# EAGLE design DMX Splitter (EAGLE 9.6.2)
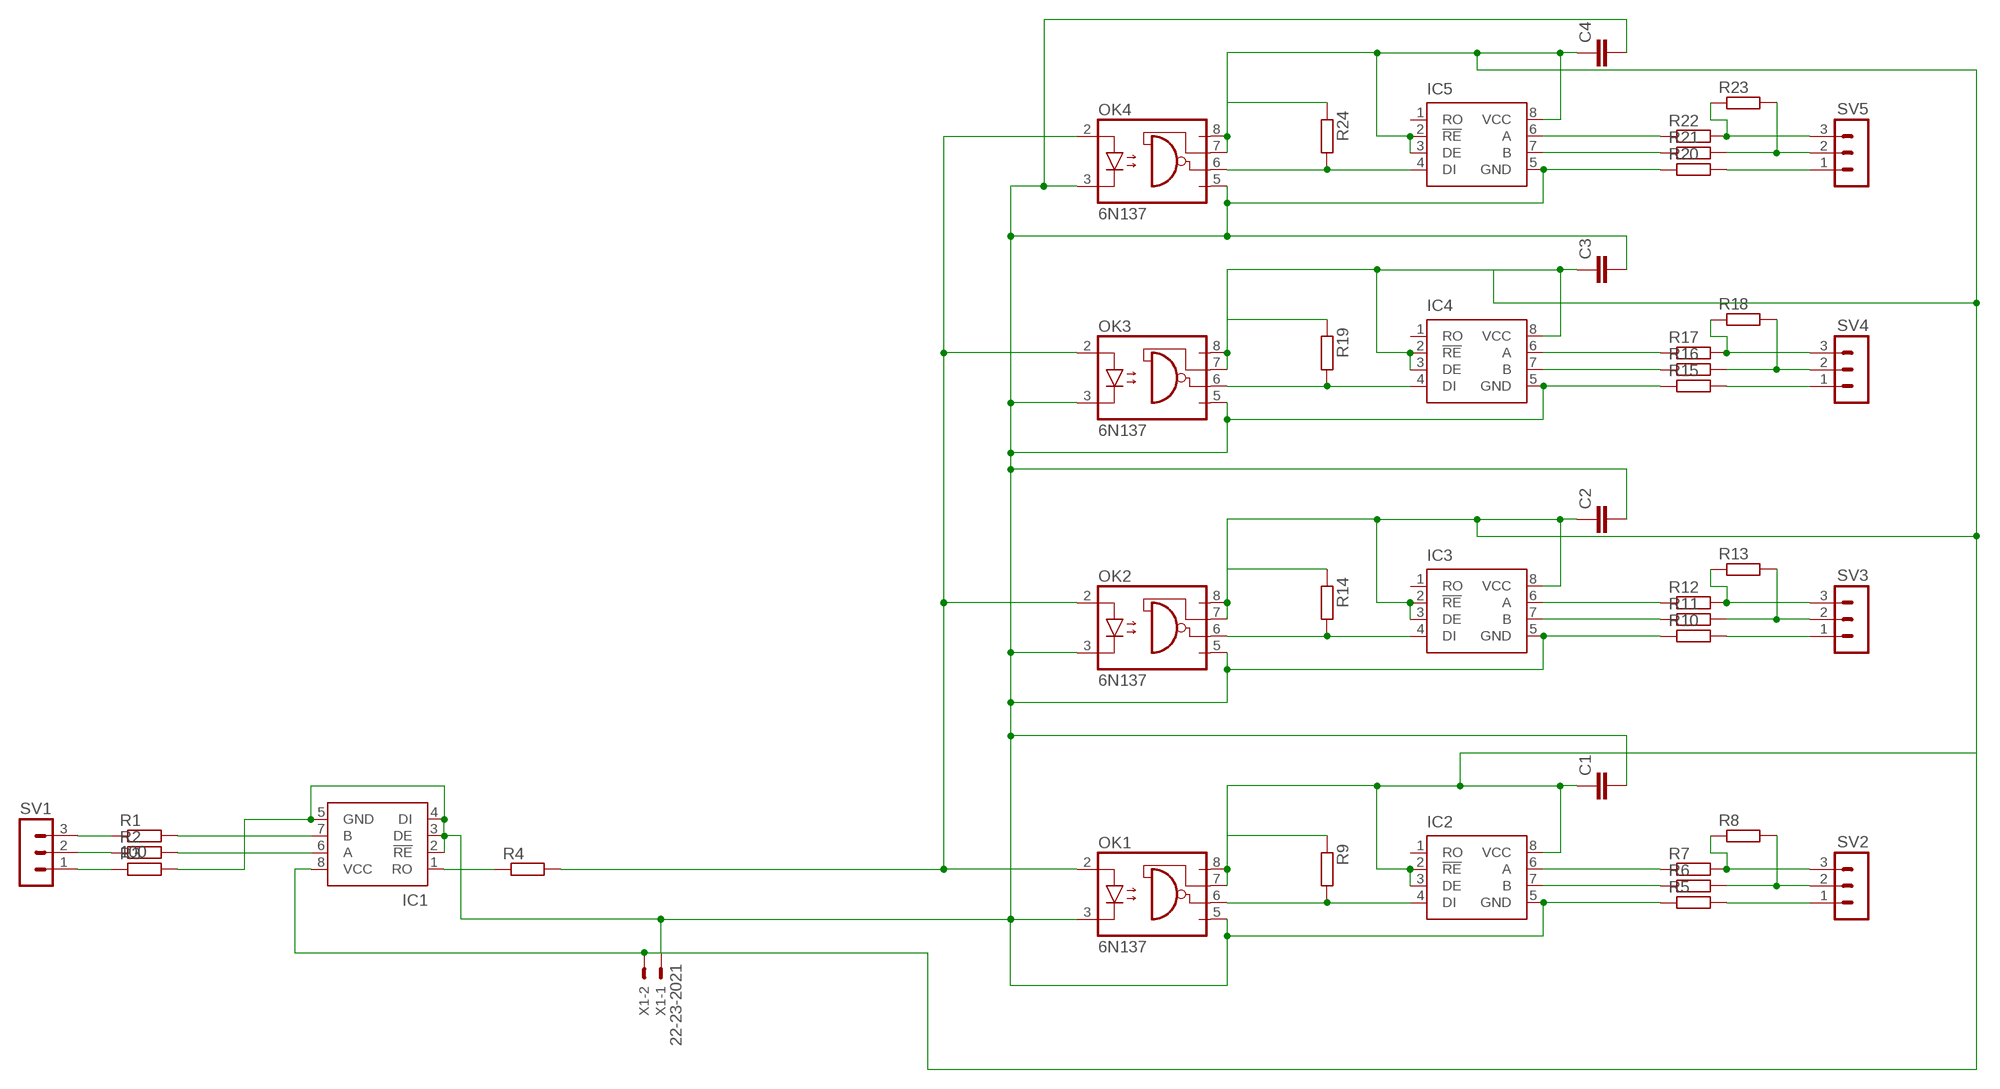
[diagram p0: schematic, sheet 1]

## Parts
C1  C-EUC025_050-024X070  [C025_050-024X070]
C2  C-EUC025_050-024X070  [C025_050-024X070]
C3  C-EUC025_050-024X070  [C025_050-024X070]
C4  C-EUC025_050-024X070  [C025_050-024X070]
IC1  LTC485N  [DIL08]
IC2  LTC485N  [DIL08]
IC3  LTC485N  [DIL08]
IC4  LTC485N  [DIL08]
IC5  LTC485N  [DIL08]
OK1  6N137  [DIL08]
OK2  6N137  [DIL08]
OK3  6N137  [DIL08]
OK4  6N137  [DIL08]
R1  100  R-EU_0207/2V  [0207/2V]
R2  R-EU_0207/2V  [0207/2V]
R3  R-EU_0207/2V  [0207/2V]
R4  R-EU_0207/2V  [0207/2V]
R5  R-EU_0207/2V  [0207/2V]
R6  R-EU_0207/2V  [0207/2V]
R7  R-EU_0207/2V  [0207/2V]
R8  R-EU_0207/2V  [0207/2V]
R9  R-EU_0207/2V  [0207/2V]
R10  R-EU_0207/2V  [0207/2V]
R11  R-EU_0207/2V  [0207/2V]
R12  R-EU_0207/2V  [0207/2V]
R13  R-EU_0207/2V  [0207/2V]
R14  R-EU_0207/2V  [0207/2V]
R15  R-EU_0207/2V  [0207/2V]
R16  R-EU_0207/2V  [0207/2V]
R17  R-EU_0207/2V  [0207/2V]
R18  R-EU_0207/2V  [0207/2V]
R19  R-EU_0207/2V  [0207/2V]
R20  R-EU_0207/2V  [0207/2V]
R21  R-EU_0207/2V  [0207/2V]
R22  R-EU_0207/2V  [0207/2V]
R23  R-EU_0207/2V  [0207/2V]
R24  R-EU_0207/2V  [0207/2V]
SV1  MA03-1  [MA03-1]
SV2  MA03-1  [MA03-1]
SV3  MA03-1  [MA03-1]
SV4  MA03-1  [MA03-1]
SV5  MA03-1  [MA03-1]
X1  22-23-2021  [22-23-2021]

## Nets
N$1: R1.1 SV1.3
N$2: R2.1 SV1.2
N$3: R3.1 SV1.1
N$4: IC1.7(B) R1.2
N$5: IC1.6(A) R2.2
N$7: IC1.1(RO) R4.1
N$9: IC2.4(DI) OK1.6(VO) R9.2
N$11: C1.1 IC2.2(!RE) IC2.3(DE) IC2.8(VCC) OK1.7(VE) OK1.8(VCC) R9.1
N$12: R7.2 R8.1 SV2.3
N$13: IC2.6(A) R7.1
N$14: R6.2 R8.2 SV2.2
N$15: R5.2 SV2.1
N$16: IC2.7(B) R6.1
N$18: IC3.4(DI) OK2.6(VO) R14.2
N$19: C2.1 C3.1 C4.1 IC1.8(VCC) IC3.2(!RE) IC3.3(DE) IC3.8(VCC) IC4.2(!RE) IC4.3(DE) IC4.8(VCC) IC5.2(!RE) IC5.3(DE) IC5.8(VCC) OK2.7(VE) OK2.8(VCC) OK3.7(VE) OK3.8(VCC) OK4.7(VE) OK4.8(VCC) R14.1 R19.1 R24.1 X1.2
N$21: R12.2 R13.1 SV3.3
N$22: IC3.6(A) R12.1
N$23: R11.2 R13.2 SV3.2
N$24: R10.2 SV3.1
N$25: IC3.7(B) R11.1
N$26: IC4.4(DI) OK3.6(VO) R19.2
N$29: R17.2 R18.1 SV4.3
N$30: IC4.6(A) R17.1
N$31: R16.2 R18.2 SV4.2
N$32: R15.2 SV4.1
N$33: IC4.7(B) R16.1
N$34: IC5.4(DI) OK4.6(VO) R24.2
N$37: R22.2 R23.1 SV5.3
N$38: IC5.6(A) R22.1
N$39: R21.2 R23.2 SV5.2
N$40: R20.2 SV5.1
N$41: IC5.7(B) R21.1
N$42: OK1.2(A) OK2.2(A) OK3.2(A) OK4.2(A) R4.2
N$44: C1.2 C2.2 C3.2 C4.2 IC1.2(!RE) IC1.3(DE) IC1.4(DI) IC1.5(GND) IC2.5(GND) IC3.5(GND) IC4.5(GND) IC5.5(GND) OK1.3(C) OK1.5(GND) OK2.3(C) OK2.5(GND) OK3.3(C) OK3.5(GND) OK4.3(C) OK4.5(GND) R3.2 R5.1 R10.1 R15.1 R20.1 X1.1
Unconnected: IC2.1(RO) IC3.1(RO) IC4.1(RO) IC5.1(RO)

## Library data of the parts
C1-C4 = rcl:C-EU: CAPACITOR, European symbol; SPICEPREFIX: C
IC1-IC5 = linear-technology:LTC485: Low Power RS485 Interface Transceiver Source: http://www.linear.com/pc/downloadDocument.do?navId=H0,C1,C1007,C1017,P2064,D1718; OC_FARNELL: unknown; OC_NEWARK: unknown
OK1-OK4 = optocoupler:6N137: MOTOROLA OPTO COUPLER; MPN: 6N137; OC_FARNELL: 1328376; OC_NEWARK: 52M1895
R1-R24 = rcl:R-EU_: RESISTOR, European symbol; SPICEPREFIX: R
SV1-SV5 = con-lstb:MA03-1: PIN HEADER; OC_FARNELL: unknown; OC_NEWARK: unknown
X1 = con-molex:22-23-2021: .100" (2.54mm) Center Header - 2 Pin; MF: MOLEX; MPN: 22-23-2021; OC_FARNELL: 1462926; OC_NEWARK: 25C3832

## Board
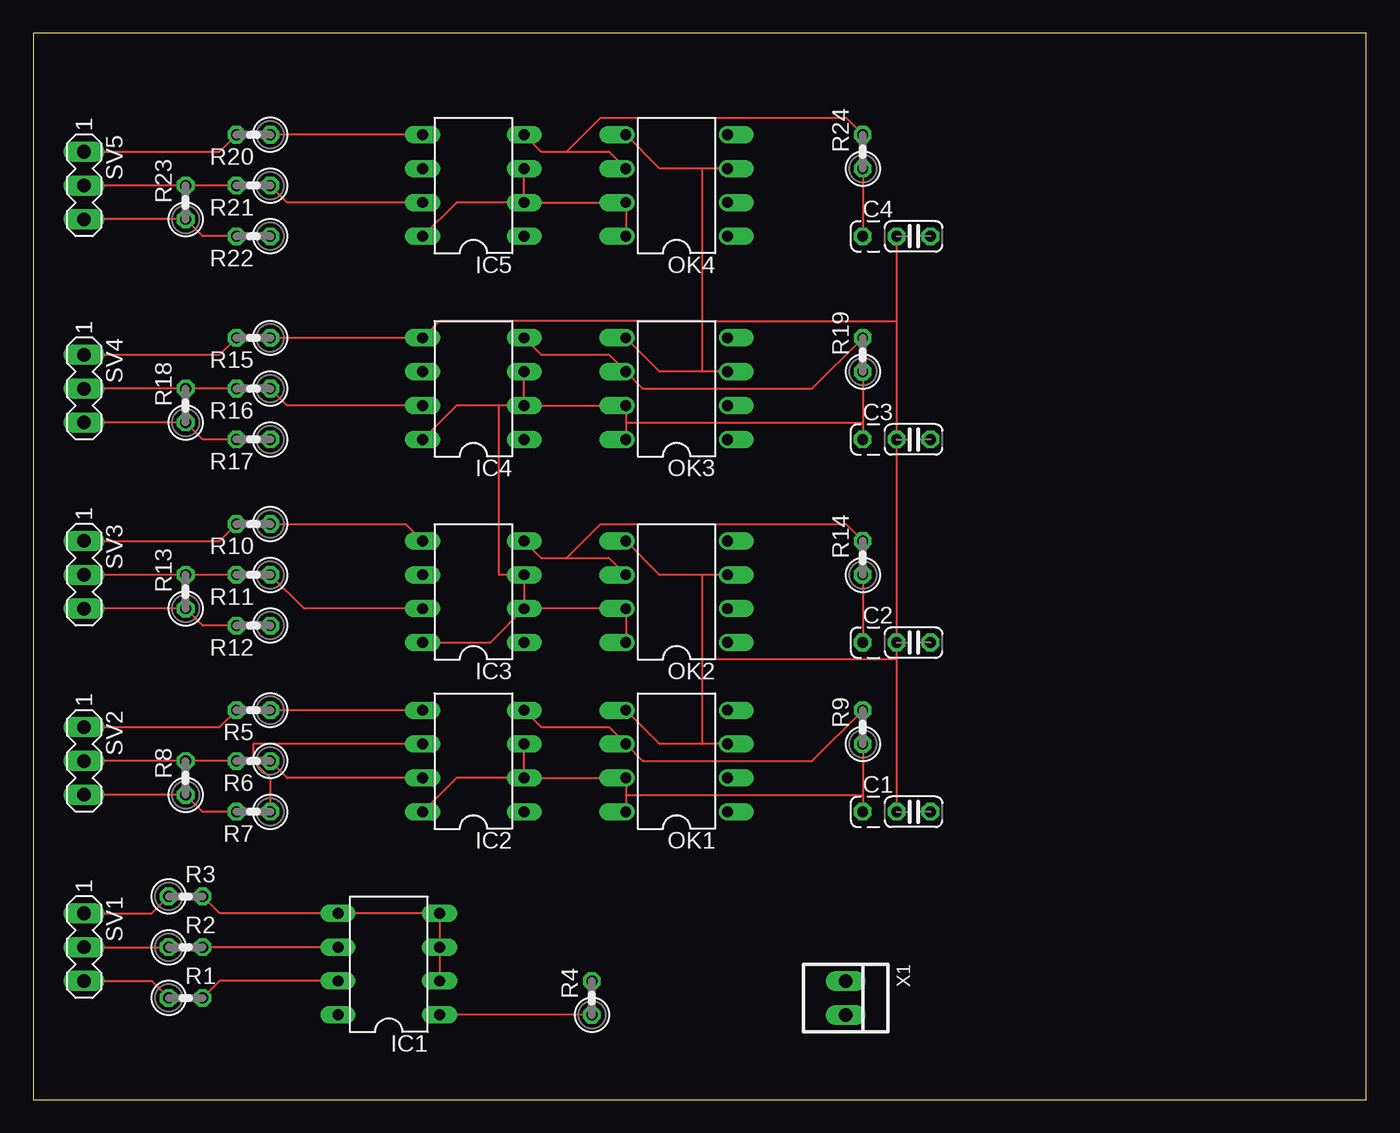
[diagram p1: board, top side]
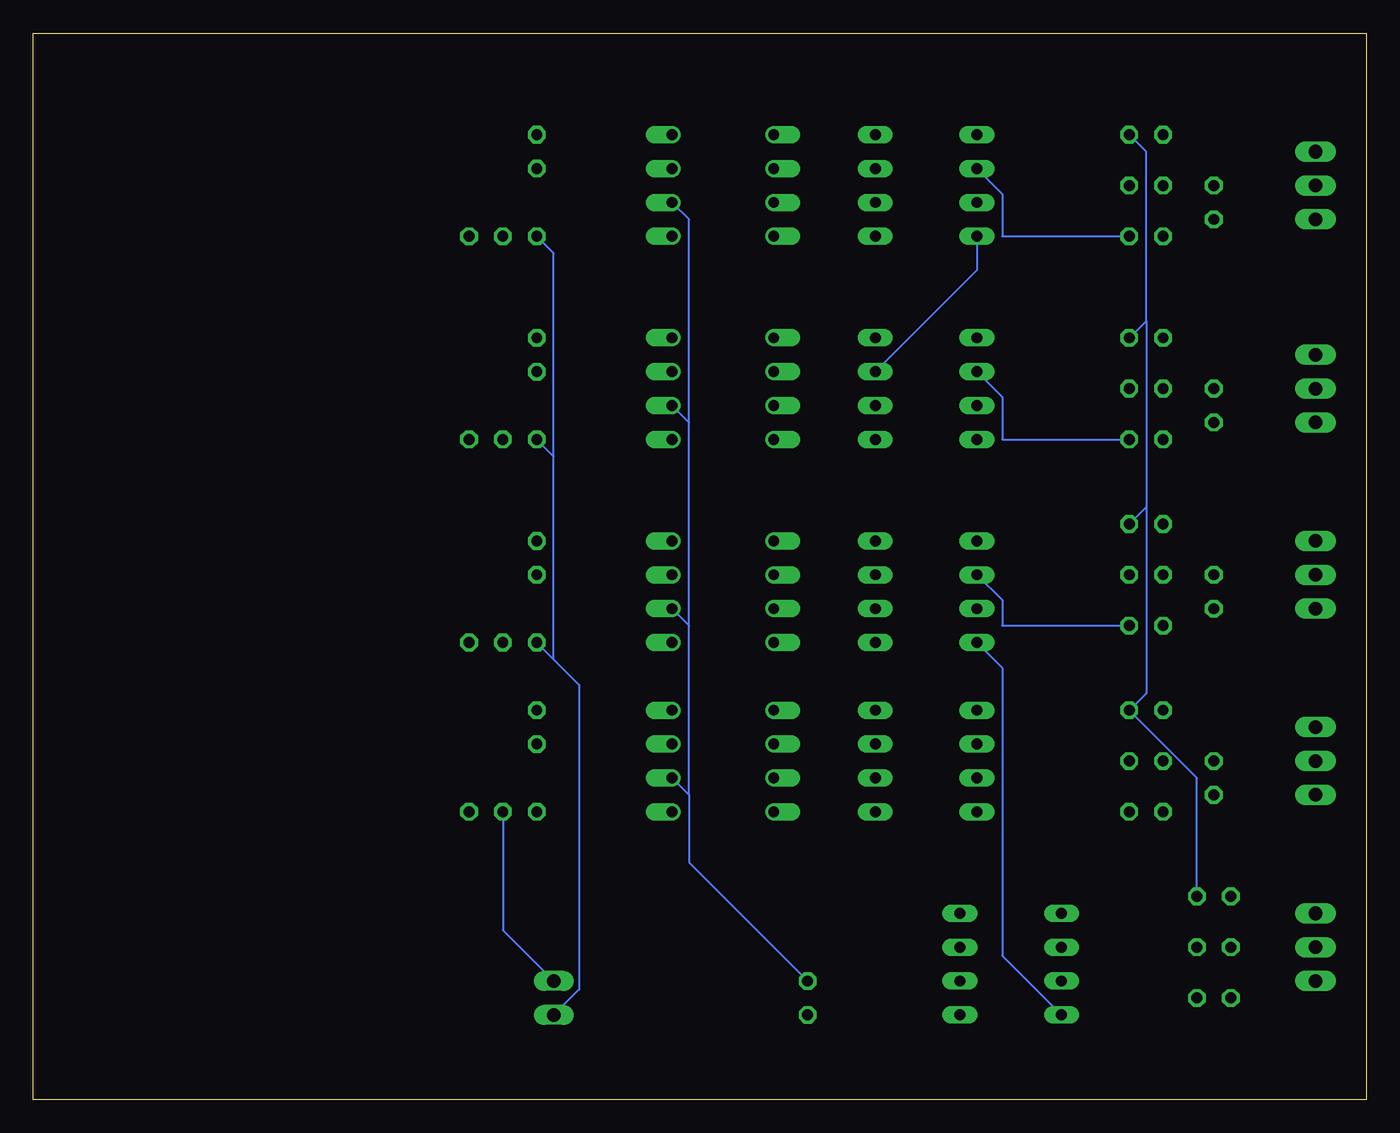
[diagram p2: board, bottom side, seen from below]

Size 100 x 80 mm. Coordinates in mm from the lower left corner, seen from the top.
Outline: 0,0 100,0 100,80 0,80 0,0
Copper layers (1*16): Top 0.035mm / dielectric 1.5mm / Bottom 0.035mm
Design rules "default": minimum track width 6mil, minimum drill 0.35mm, track to track 6mil, track to pad 6mil, pad to pad 6mil, via to via 6mil, smd to smd 6mil, copper to edge 40mil, drill to drill 6mil, minimum pad ring 10mil, minimum via ring 8mil, stop-mask expansion 4mil, vias tented up to drill 0mil, thermal gap 10mil

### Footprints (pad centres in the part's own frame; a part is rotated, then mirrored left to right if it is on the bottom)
C025_050-024X070 = drill 0.813 octagon: 1 -3.81,0; 2 -1.27,0; 3 1.27,0
DIL08 = drill 0.813 long: 1 -3.81,-3.81; 2 -1.27,-3.81; 3 1.27,-3.81; 4 3.81,-3.81; 5 3.81,3.81; 6 1.27,3.81; 7 -1.27,3.81; 8 -3.81,3.81
DIL08' = drill 0.813 offset: 1 -3.81,-3.81; 2 -1.27,-3.81; 3 1.27,-3.81; 4 3.81,-3.81; 5 3.81,3.81; 6 1.27,3.81; 7 -1.27,3.81; 8 -3.81,3.81
0207/2V = drill 0.813 octagon: 1 -1.27,0; 2 1.27,0
MA03-1 = drill 1.016 long: 1 -2.54,0; 2 0,0; 3 2.54,0
22-23-2021 = drill 1 long: 1 -1.27,0; 2 1.27,0

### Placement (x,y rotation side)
C1  66.04,21.59 0 top
C2  66.04,34.29 0 top
C3  66.04,49.53 0 top
C4  66.04,64.77 0 top
IC1  26.67,10.16 90 top
IC2  33.02,25.4 90 top
IC3  33.02,38.1 90 top
IC4  33.02,53.34 90 top
IC5  33.02,68.58 90 top
OK1  6N137  [DIL08']  48.26,25.4 90 top
OK2  6N137  [DIL08']  48.26,38.1 90 top
OK3  6N137  [DIL08']  48.26,53.34 90 top
OK4  6N137  [DIL08']  48.26,68.58 90 top
R1  [0207/2V]  11.43,7.62 0 top
R2  11.43,11.43 0 top
R3  11.43,15.24 0 top
R4  41.91,7.62 90 top
R5  16.51,29.21 180 top
R6  16.51,25.4 180 top
R7  16.51,21.59 180 top
R8  11.43,24.13 90 top
R9  62.23,27.94 90 top
R10  16.51,43.18 180 top
R11  16.51,39.37 180 top
R12  16.51,35.56 180 top
R13  11.43,38.1 90 top
R14  62.23,40.64 90 top
R15  16.51,57.15 180 top
R16  16.51,53.34 180 top
R17  16.51,49.53 180 top
R18  11.43,52.07 90 top
R19  62.23,55.88 90 top
R20  16.51,72.39 180 top
R21  16.51,68.58 180 top
R22  16.51,64.77 180 top
R23  11.43,67.31 90 top
R24  62.23,71.12 90 top
SV1  3.81,11.43 270 top
SV2  3.81,25.4 270 top
SV3  3.81,39.37 270 top
SV4  3.81,53.34 270 top
SV5  3.81,68.58 270 top
X1  60.96,7.62 270 top

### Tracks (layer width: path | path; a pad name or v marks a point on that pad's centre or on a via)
N$1
  Top 0.152: R1.1 8.89,8.89 SV1.3
N$2
  Top 0.152: SV1.2 R2.1
N$3
  Top 0.152: R3.1 8.89,13.97 SV1.1
N$4
  Top 0.152: R1.2 13.97,8.89 IC1.7
N$5
  Top 0.152: IC1.6 R2.2
N$7
  Top 0.152: R4.1 IC1.1
N$9
  Top 0.152: IC2.4 38.1,27.94 43.18,27.94 OK1.6 45.72,25.4 58.42,25.4 R9.2
N$11
  Top 0.152: R9.1 62.23,22.86 | 62.23,22.86 C1.1 | 44.45,22.86 OK1.7 IC2.2 | 44.45,22.86 OK1.8 | IC2.8 31.75,24.13 IC2.2 | IC2.2 IC2.3 | 44.45,22.86 62.23,22.86
N$12
  Top 0.152: R7.2 12.7,21.59 R8.1 SV2.3
N$13
  Top 0.152: R7.1 17.78,24.13 16.51,25.4 16.51,26.67 IC2.6
N$14
  Top 0.152: R6.2 R8.2 SV2.2
N$15
  Top 0.152: R5.2 13.97,27.94 SV2.1
N$16
  Top 0.152: R6.1 19.05,24.13 IC2.7
N$18
  Top 0.152: OK2.6 43.18,40.64 40.01,40.64 | 40.01,40.64 38.1,40.64 IC3.4 | R14.2 60.96,43.18 42.55,43.18 40.01,40.64
N$19
  Top 0.152: R24.1 C4.1 | R19.1 62.23,50.8 | 62.23,50.8 C3.1 | R14.1 C2.1 | 44.45,50.8 OK3.7 IC4.2 | 44.45,50.8 OK3.8 | IC4.8 31.75,52.07 34.92,52.07 | IC4.2 34.92,52.07 | IC4.2 IC4.3 | OK4.8 OK4.7 IC5.2 | IC5.8 31.75,67.31 IC5.2 | IC5.2 IC5.3 | IC3.2 IC3.3 34.92,39.37 34.92,52.07 | OK2.8 OK2.7 IC3.2 | IC3.2 34.29,34.29 IC3.8 | 44.45,50.8 62.23,50.8
  Bottom 0.152: X1.2 59.05,8.26 59.05,31.11 60.96,33.02 | C2.1 60.96,33.02 | 60.96,48.26 C3.1 | 60.96,33.02 60.96,48.26 | C4.1 60.96,63.5 60.96,48.26 | IC4.3 29.21,62.23 IC5.8 | IC1.8 27.3,10.79 27.3,32.38 IC3.8
N$21
  Top 0.152: R12.2 12.7,35.56 R13.1 SV3.3
N$22
  Bottom 0.152: R12.1 27.3,35.56 27.3,37.47 IC3.6
N$23
  Top 0.152: R11.2 R13.2 SV3.2
N$24
  Top 0.152: R10.2 13.97,41.91 SV3.1
N$25
  Top 0.152: R11.1 20.32,36.83 IC3.7
N$26
  Top 0.152: IC4.4 38.1,55.88 43.18,55.88 OK3.6 45.72,53.34 58.42,53.34 R19.2
N$29
  Top 0.152: R17.2 12.7,49.53 R18.1 SV4.3
N$30
  Bottom 0.152: R17.1 27.3,49.53 27.3,52.7 IC4.6
N$31
  Top 0.152: R16.2 R18.2 SV4.2
N$32
  Top 0.152: R15.2 13.97,55.88 SV4.1
N$33
  Top 0.152: R16.1 19.05,52.07 IC4.7
N$34
  Top 0.152: OK4.6 43.18,71.12 40.01,71.12 | 40.01,71.12 38.1,71.12 IC5.4 | R24.2 60.96,73.66 42.55,73.66 40.01,71.12
N$37
  Top 0.152: R22.2 12.7,64.77 R23.1 SV5.3
N$38
  Bottom 0.152: R22.1 27.3,64.77 27.3,67.94 IC5.6
N$39
  Top 0.152: R21.2 R23.2 SV5.2
N$40
  Top 0.152: R20.2 13.97,71.12 SV5.1
N$41
  Top 0.152: R21.1 19.05,67.31 IC5.7
N$42
  Bottom 0.152: R4.2 50.8,17.78 50.8,22.86 | OK1.2 50.8,22.86 | 50.8,35.56 OK2.2 | 50.8,22.86 50.8,35.56 | 50.8,50.8 OK3.2 | 50.8,35.56 50.8,50.8 | OK4.2 50.8,66.04 50.8,50.8
N$44
  Top 0.152: OK1.5 46.99,26.67 50.16,26.67 | OK1.3 50.16,26.67 | OK2.5 46.99,39.37 50.16,39.37 | OK2.3 50.16,39.37 | 50.16,39.37 50.16,33.02 | 50.16,33.02 50.16,26.67 | 64.77,33.02 C2.2 C3.2 64.77,58.42 | 64.77,33.02 C1.2 | 64.77,33.02 50.16,33.02 | IC2.5 R5.1 | IC1.2 IC1.3 IC1.4 IC1.5 13.97,13.97 R3.2 | C4.2 64.77,58.42 | IC3.5 27.94,43.18 R10.1 | IC5.5 R20.1 | R15.1 IC4.5 30.48,58.42 50.16,58.42 | OK3.5 46.99,54.61 50.16,54.61 | OK3.3 50.16,54.61 | OK4.5 46.99,69.85 50.16,69.85 | OK4.3 50.16,69.85 | 50.16,69.85 50.16,58.42 | 50.16,58.42 50.16,54.61 | 50.16,58.42 64.77,58.42
  Bottom 0.152: X1.1 64.77,12.7 C1.2 | R3.2 12.7,24.13 R5.1 16.51,30.48 16.51,44.45 | R20.1 16.51,71.12 16.51,58.42 | R15.1 16.51,58.42 | 16.51,44.45 R10.1 | 16.51,58.42 16.51,44.45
